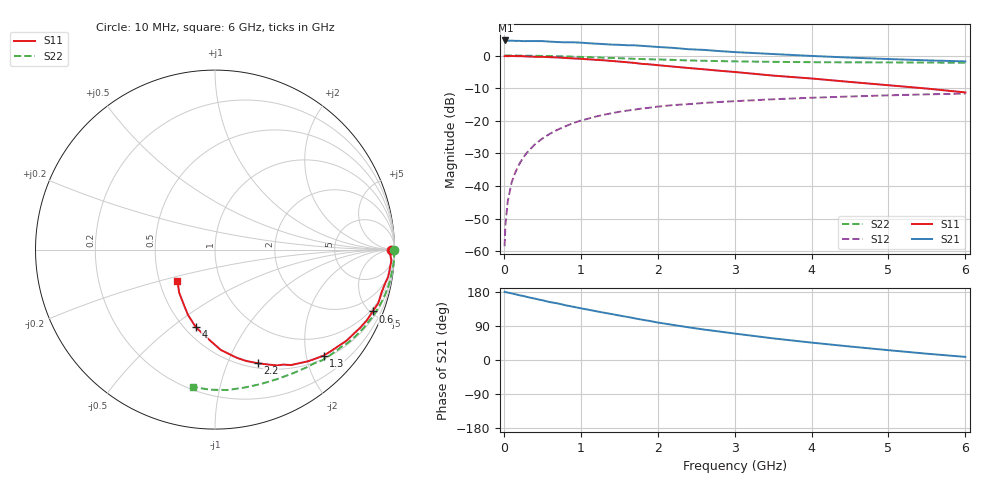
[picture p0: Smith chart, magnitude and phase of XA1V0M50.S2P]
! SIEMENS Discrete & RF Semiconductors
! BFY180
! Si NPN RF Bipolar Junction Transistor in MICRO-X
! VCE = 1 V  IC = 0.5 mA
! Common Emitter S-Parameters:  May  1997
# GHz  S  MA  R  50
!  f  S11  S21  S12  S22
! GHz  MAG  ANG  MAG  ANG  MAG  ANG  MAG  ANG
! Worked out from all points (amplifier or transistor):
!   36 points, 10 MHz to 6 GHz, reference 50 ohm
!   highest |S21| = 4.6 dB at 20 MHz (marker M1)
!   |S21| within 3 dB of that: start of sweep to 2.661 GHz
!   unconditionally stable (mu >= 1): 4.371 GHz to end of sweep
!   at 250 MHz: K = 0.06, MSG = 17.9 dB, |S12| = -31.3 dB
!   at 1.4 GHz: K = 0.44, MSG = 10.5 dB, |S12| = -17.7 dB
!   at 6 GHz: K = 1.07, MAG = 3.4 dB, |S12| = -11.7 dB
!   S11 on the Smith chart (normalised r, x): 10 MHz: 88, -14; 600 MHz: 0.82, -5.17; 1.3 GHz: 0.56, -2.34; 2.2 GHz: 0.55, -1.29; 4 GHz: 0.57, -0.61; 6 GHz: 0.62, -0.23
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0.01  0.978 -0.2  1.681 179.9  0.0012 77.0  0.9978 -0.2
0.02  0.9844 -0.8  1.703 179.0  0.0025 97.2  0.9989 -0.4
0.05  0.9776 -1.8  1.681 178.0  0.0057 87.5  0.9991 -1.2
0.1  0.9845 -3.6  1.694 175.8  0.0113 88.2  0.999 -2.5
0.2  0.9789 -7.2  1.68 171.0  0.0216 84.8  0.9968 -4.8
0.3  0.9681 -10.8  1.666 166.5  0.0324 81.4  0.9936 -7.2
0.4  0.9583 -14.3  1.667 162.0  0.0432 79.6  0.991 -9.6
0.5  0.9574 -18.2  1.665 157.6  0.0535 76.2  0.987 -12.0
0.6  0.9435 -21.4  1.634 152.7  0.0634 73.5  0.9814 -14.3
0.9  0.903 -31.5  1.595 140.6  0.092 65.5  0.961 -21.1
1.1  0.8747 -37.6  1.545 132.6  0.1082 60.4  0.9437 -25.5
1.3  0.8456 -44.3  1.497 124.9  0.1239 55.6  0.9273 -29.7
1.7  0.7704 -56.6  1.434 110.0  0.1485 47.4  0.8897 -37.3
2  0.7121 -64.3  1.354 98.9  0.1649 42.0  0.8704 -42.5
2.2  0.6772 -69.3  1.311 92.6  0.1741 38.3  0.8584 -46.0
2.6  0.6156 -78.5  1.221 80.4  0.1877 32.6  0.8319 -51.9
3  0.56 -86.7  1.13 69.8  0.1998 27.3  0.8146 -57.7
3.5  0.4929 -95.3  1.055 57.1  0.2139 22.1  0.8003 -64.4
4  0.4451 -103.9  0.986 45.9  0.2256 16.7  0.7914 -71.1
4.5  0.3943 -112.4  0.93 35.6  0.2357 12.0  0.7861 -78.0
5.5  0.3119 -129.8  0.844 16.6  0.2545 2.5  0.7813 -92.0
6  0.272 -140.4  0.813 8.2  0.2611 -2.2  0.7747 -99.1
